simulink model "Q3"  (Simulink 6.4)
settings: Solver=ode4  StartTime=0.0  StopTime=10  FixedStep=0.01  RelTol=1e-3
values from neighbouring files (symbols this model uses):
  A = pi*R^2    (= 0.0669661890039)    [par.m]
  a = 14    [par.m]
  Cd = 0.02    [par.m]
  Cd_sfe = 0.24    [par.m]
  g = 9.81    [par.m]
  h = -0.012    [par.m]
  I = diag([Ix Iy Iz])    [par.m]
  I_inv = inv(I)    [par.m]
  J = Ja+Jr/(n^2)    (= 2.07047193878e-06)    [par.m]
  Ja = 1e-006    (= 1e-06)    [par.m]
  Jr = 3.357e-005    (= 3.357e-05)    [par.m]
  K = 0.00345    [par.m]
  l = 0.237    [par.m]
  m = 0.488    [par.m]
  Minv = inv(M)    [par.m]
  n = 5.6    [par.m]
  omegah = x    (= 300)    [par.m]
  r = 0.1    [par.m]
  R = 0.146    [par.m]
  rho = 1.225    [par.m]
  s = b*c*R/A    (= 0.100289416195)    [par.m]
  tau = Ra*J/K^2    (= 0.22300735354)    [par.m]
  teta = 0.22    [par.m]
  x0 = []    [betaDx.m]    (also in alfa.m; control.m = zeros(16,1); beta.m; lambda.m)
libraries: aerolibutil x11, simulink x8, aerosimlib x8
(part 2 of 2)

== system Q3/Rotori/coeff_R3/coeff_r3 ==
  note: [p_ad q_ad r_ad mu lambda chi]
  in_coeff : Inport
  Mux2 : Mux  Inputs=5
  hc : Fcn  Expr=1/4*Cd*u(4)*(u(6)-u(3))+1/12*a*(-teta*u(6)*u(1)+teta*u(3)*u(1)-3*u(5)*u(1)-3*teta*u(4)*u(5))
  pc : Fcn  Expr=1/16*a*u(2)*(u(3)-u(6))
  qc : Fcn  Expr=1/8*Cd*(u(6)^2+u(3)^2-2*u(6)*u(3)+u(4)^2)+1/48*a*(-3*u(1)^2-3*u(2)^2-4*teta*u(4)*u(1)+8*teta*u(3)*u(5)-8*teta*u(6)*u(5)-12*u(5)^2)
  rc : Fcn  Expr=-1/48*a*(u(4)*(8*teta*u(3)-8*u(6)*teta-6*u(5))+3*u(1)*(u(3)-u(6)))
  tc : Fcn  Expr=1/24*a*(teta*(4*u(6)^2-8*u(6)*u(3)+4*u(3)^2+6*u(4)^2)+6*u(5)*(u(6)-u(3))+3*u(4)*u(1))
  coeff3 : Outport
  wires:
  in_coeff/1 -> qc/1, rc/1, pc/1, hc/1, tc/1
  tc/1 -> Mux2/1
  hc/1 -> Mux2/2
  Mux2/1 -> coeff3/1
  qc/1 -> Mux2/3
  rc/1 -> Mux2/4
  pc/1 -> Mux2/5

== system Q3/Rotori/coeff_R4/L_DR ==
  betax : Inport
  Constant : Constant  Value=0  OutDataType=sfix(16)  ConRadixGroup=Use specified scaling  OutScaling=2^0  SampleTime=inf  FramePeriod=inf
  Constant1 : Constant  Value=1  OutDataType=sfix(16)  ConRadixGroup=Use specified scaling  OutScaling=2^0  SampleTime=inf  FramePeriod=inf
  Gain : Gain  Gain=-1
  Matrix Concatenation : Concatenate  NumInputs=3  Mode=Horizontal matrix concatenation
  Matrix Concatenation1 : Concatenate  NumInputs=3  Mode=Horizontal matrix concatenation
  Matrix Concatenation2 : Concatenate  NumInputs=3  Mode=Horizontal matrix concatenation
  Matrix Concatenation3 : Concatenate  NumInputs=3  Mode=Vertical matrix concatenation
  sin(beta) : Trigonometry
  sin(beta)1 : Trigonometry  Operator=cos
  L_DR : Outport
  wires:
  Matrix Concatenation3/1 -> L_DR/1
  Matrix Concatenation2/1 -> Matrix Concatenation3/3
  Matrix Concatenation1/1 -> Matrix Concatenation3/2
  Matrix Concatenation/1 -> Matrix Concatenation3/1
  Constant1/1 -> Matrix Concatenation2/3
  Constant/1 -> Matrix Concatenation2/2, Matrix Concatenation2/1, Matrix Concatenation1/3, Matrix Concatenation/3
  sin(beta)/1 -> Gain/1, Matrix Concatenation/2
  sin(beta)1/1 -> Matrix Concatenation1/2, Matrix Concatenation/1
  betax/1 -> sin(beta)/1, sin(beta)1/1
  Gain/1 -> Matrix Concatenation1/1

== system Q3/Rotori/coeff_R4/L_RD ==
  betax : Inport
  Constant : Constant  Value=0  OutDataType=sfix(16)  ConRadixGroup=Use specified scaling  OutScaling=2^0  SampleTime=inf  FramePeriod=inf
  Constant1 : Constant  Value=1  OutDataType=sfix(16)  ConRadixGroup=Use specified scaling  OutScaling=2^0  SampleTime=inf  FramePeriod=inf
  Gain : Gain  Gain=-1
  Matrix Concatenation : Concatenate  NumInputs=3  Mode=Horizontal matrix concatenation
  Matrix Concatenation1 : Concatenate  NumInputs=3  Mode=Horizontal matrix concatenation
  Matrix Concatenation2 : Concatenate  NumInputs=3  Mode=Horizontal matrix concatenation
  Matrix Concatenation3 : Concatenate  NumInputs=3  Mode=Vertical matrix concatenation
  sin(beta) : Trigonometry
  sin(beta)1 : Trigonometry  Operator=cos
  L_RD4 : Outport
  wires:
  Matrix Concatenation3/1 -> L_RD4/1
  Matrix Concatenation2/1 -> Matrix Concatenation3/3
  Matrix Concatenation1/1 -> Matrix Concatenation3/2
  Matrix Concatenation/1 -> Matrix Concatenation3/1
  Constant1/1 -> Matrix Concatenation2/3
  Constant/1 -> Matrix Concatenation2/2, Matrix Concatenation2/1, Matrix Concatenation1/3, Matrix Concatenation/3
  Gain/1 -> Matrix Concatenation/2
  sin(beta)/1 -> Matrix Concatenation1/1, Gain/1
  sin(beta)1/1 -> Matrix Concatenation1/2, Matrix Concatenation/1
  betax/1 -> sin(beta)/1, sin(beta)1/1

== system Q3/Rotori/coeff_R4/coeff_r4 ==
  note: [p_ad q_ad r_ad mu lambda chi]
  in_coeff : Inport
  Mux2 : Mux  Inputs=5
  hc : Fcn  Expr=1/4*Cd*u(4)*(u(6)+u(3))+1/12*a*(teta*u(6)*u(1)+teta*u(3)*u(1)+3*u(5)*u(1)-3*teta*u(4)*u(5))
  pc : Fcn  Expr=-1/16*a*u(2)*(u(3)+u(6))
  qc : Fcn  Expr=1/8*Cd*(u(6)^2+u(3)^2+2*u(6)*u(3)+u(4)^2)+1/48*a*(-3*u(1)^2-3*u(2)^2+4*teta*u(4)*u(1)-8*teta*u(3)*u(5)-8*teta*u(6)*u(5)-12*u(5)^2)
  rc : Fcn  Expr=-1/48*a*(u(4)*(-8*teta*u(3)-8*u(6)*teta-6*u(5))+3*u(1)*(u(3)+u(6)))
  tc : Fcn  Expr=1/24*a*(teta*(4*u(6)^2+8*u(6)*u(3)+4*u(3)^2+6*u(4)^2)+6*u(5)*(u(6)+u(3))-3*u(4)*u(1))
  coeff4 : Outport
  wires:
  in_coeff/1 -> qc/1, rc/1, pc/1, hc/1, tc/1
  tc/1 -> Mux2/1
  hc/1 -> Mux2/2
  Mux2/1 -> coeff4/1
  qc/1 -> Mux2/3
  rc/1 -> Mux2/4
  pc/1 -> Mux2/5
